DATA_BLOCK DB 1
STRUCT
	DT1	: DATE_AND_TIME;
	DT2	: DATE_AND_TIME;
	DT3	: DATE_AND_TIME;
END_STRUCT;
BEGIN
//TODO	DT1 := DT#90-1-1-0:0:0.000;
//	DT2 := DT#90-1-1-0:0:0.000;
//	DT3 := DT#90-1-1-0:0:0.000;
END_DATA_BLOCK


FUNCTION FC 1 : VOID
BEGIN
	AUF		DB 1
	LAR1		P#DBX 0.0

	// Rotate DB1.DT1 one bit to the left
	L		D [AR1,P#4.0]
	UD		DW#16#80000000
	L		D [AR1,P#0.0]
	RLDA
	T		D [AR1,P#0.0]
	L		D [AR1,P#4.0]
	RLDA
	T		D [AR1,P#4.0]

	// Rotate DB1.DT2 one bit to the left
	L		D [AR1,P#12.0]
	UD		DW#16#80000000
	L		D [AR1,P#8.0]
	RLDA
	T		D [AR1,P#8.0]
	L		D [AR1,P#12.0]
	RLDA
	T		D [AR1,P#12.0]

	// Compare DB1.DT1 to DB1.DT2
	// Should be equal
	CALL "EQ_DT" (
		DT1	:= DB1.DT1,
		DT2	:= DB1.DT2,
		RET_VAL	:= M 0.0,
	)
	U		M 0.0
	__ASSERT==	__STW VKE,	1

	// Compare DB1.DT1 to DB1.DT3
	// Should be not equal
	CALL "EQ_DT" (
		DT1	:= DB1.DT1,
		DT2	:= DB1.DT3,
		RET_VAL	:= M 0.1,
	)
	U		M 0.1
	__ASSERT==	__STW VKE,	0

	// Decrement the test counter.
	// Stop test, if it reaches zero.
	U		DBX 0.0
	ZR		Z 0
	U		Z 0
	SPB		m003
	CALL		SFC 46 // Stop CPU
m003:	NOP		0
END_FUNCTION


ORGANIZATION_BLOCK OB 1
BEGIN
	CALL		FC 1
END_ORGANIZATION_BLOCK


ORGANIZATION_BLOCK OB 100
BEGIN
	AUF		DB 1
	LAR1		P#DBX 0.0

	// Initialize DB1.DT1 (one bit set)
	L		1
	T		D [AR1,P#0.0]
	L		0
	T		D [AR1,P#4.0]

	// Initialize DB1.DT2 (one bit set)
	L		1
	T		D [AR1,P#8.0]
	L		0
	T		D [AR1,P#12.0]

	// Initialize DB1.DT3 (all bits clear)
	L		0
	T		D [AR1,P#16.0]
	L		0
	T		D [AR1,P#20.0]

	// Initialize the test counter.
	// Run 10 test loops.
	L		C#10
	CLR
	S		Z 0
	SET
	S		Z 0
END_ORGANIZATION_BLOCK
